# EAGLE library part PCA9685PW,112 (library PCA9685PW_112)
16-channel, 12-bit PWM Fm+ I2C-bus LED controller Source: Datasheet
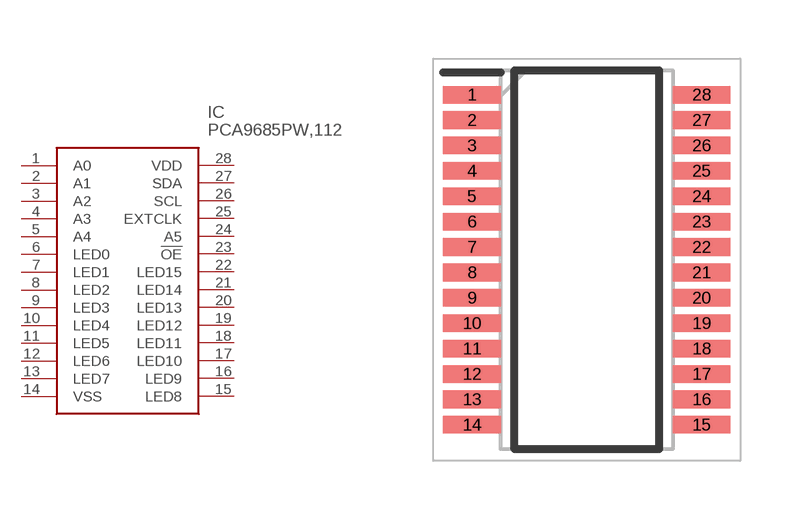
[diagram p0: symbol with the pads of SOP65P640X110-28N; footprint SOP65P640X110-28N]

Designator prefix IC

## PCA9685PW,112 (Arrow_Part_Number: PCA9685PW,112; Arrow_Price-Stock: https://www.arrow.com/en/products/pca9685pw112/nxp-semiconductors; Description: 16-channel, 12-bit PWM Fm+ I2C-bus LED controller; Height: 1.1mm; Manufacturer_Name: NXP; Manufacturer_Part_Number: PCA9685PW,112; Mouser_Part_Number: 771-PCA9685PW,112; Mouser_Price-Stock: https://www.mouser.co.uk/ProductDetail/NXP-Semiconductors/PCA9685PW112/?qs=6YAT8rHPFU9wZqiAeiOMZw%3D%3D)  [SOP65P640X110-28N]
1  A0
2  A1
3  A2
4  A3
5  A4
6  LED0
7  LED1
8  LED2
9  LED3
10  LED4
11  LED5
12  LED6
13  LED7
14  VSS
15  LED8
16  LED9
17  LED10
18  LED11
19  LED12
20  LED13
21  LED14
22  LED15
23  !OE
24  A5
25  EXTCLK
26  SCL
27  SDA
28  VDD

## Footprint SOP65P640X110-28N (pad centres in mm)
SOT361-1
smd 1.475 x 0.45: 1 -2.938,4.225; 2 -2.938,3.575; 3 -2.938,2.925; 4 -2.938,2.275; 5 -2.938,1.625; 6 -2.938,0.975; 7 -2.938,0.325; 8 -2.938,-0.325; 9 -2.938,-0.975; 10 -2.938,-1.625; 11 -2.938,-2.275; 12 -2.938,-2.925; 13 -2.938,-3.575; 14 -2.938,-4.225; 15 2.938,-4.225; 16 2.938,-3.575; 17 2.938,-2.925; 18 2.938,-2.275; 19 2.938,-1.625; 20 2.938,-0.975; 21 2.938,-0.325; 22 2.938,0.325; 23 2.938,0.975; 24 2.938,1.625; 25 2.938,2.275; 26 2.938,2.925; 27 2.938,3.575; 28 2.938,4.225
